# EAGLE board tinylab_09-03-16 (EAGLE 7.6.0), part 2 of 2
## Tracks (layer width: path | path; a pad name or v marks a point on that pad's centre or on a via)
3.3V  (via drill 0.51 pad 1.02)
  Top 0.406: 189.83,46.67 R37.2 | 189.83,40.96 R39.2 | v127.65,90.17 IC3.2 127.65,85.72
  Top 0.61: U$10.1 175.7,69.01 179.72,73.02 | Q4.1 189.83,40.96 | IC5.4 121.32,102.84 121.93,102.23 C12.A | 122.07,100.59 C12.A | 127.65,84.45 121.3,84.45 118.12,81.28 117.17,81.28 115.9,80.01 U$4.3V | 127.65,84.45 127.65,85.72 | 191.46,41.59 191.78,41.91 191.78,46.36 191.52,46.62 R37.2 189.19,47.31 187.02,47.31 186.38,46.67 Q3.1 185.7,49.26 185.43,49.53 185.43,69.21 185.7,69.48 C27.1 186.7,71.75 187.34,72.39 R42.2 R43.2 183.26,74.03 182.26,73.02 179.72,73.02 | 191.46,41.59 190.88,41.01 R39.2 | U5.4 198.06,30.41 v198.13,30.48 | 191.46,41.59 192.42,40.64 v192.42,39.37 192.1,39.05 177.49,39.05 175.27,36.83 C17.1 175.01,36.72 U$15.1 | 127.65,84.45 137.17,84.45 v140.35,87.63 | 179.72,73.02 178.13,74.61 178.13,83.5 177.49,84.14 JP8.3 JP8.5 JP8.6 171.15,86.68 170.51,86.04 170.51,82.23 171.15,81.6 JP8.2 | v127.65,100.33 127.33,100.65 125.74,100.65 125.43,100.96 124.52,100.96 C11.1 122.38,100.91 C12.A
  Bottom 0.61: v127.65,100.33 v127.65,90.17 | v198.13,30.48 198.13,35.56 196.23,37.47 194.32,37.47 v192.42,39.37 | v140.35,87.63 140.35,99.06 142.25,100.96 142.25,107.95 144.16,109.85 154.95,109.85 158.13,106.68 158.13,102.23 160.67,99.69 166.38,99.69 168.92,97.16 168.92,75.67 U$10.1
4  (via drill 0.51 pad 1.02, 0.6)
  Top 0.406: S11.4 156.22,62.23 U$4.D4 v144.79,62.23 | U$1.25 126.24,77.01 126.69,77.47 131.46,77.47 v132.09,76.83
  Bottom 0.406: v144.79,62.23 141.93,62.23 140.35,63.82 138.12,63.82 137.81,64.14 137.81,76.52 136.86,77.47 132.73,77.47 v132.09,76.83
5  (via drill 0.51 pad 1.02, 0.6)
  Top 0.406: U$1.31 121.44,81.42 122.57,82.55 135.27,82.55 135.9,81.91 135.9,80.64 136.54,80.01 139.08,80.01 v139.71,80.64 | S11.3 156.22,64.77 U$4.D5 v144.79,64.77
  Bottom 0.406: v139.71,80.64 139.71,78.74 139.08,78.1 139.08,65.41 139.71,64.77 v144.79,64.77
6
  Top 0.406: U$1.27 124.64,79.54 125.11,80.01 132.73,80.01 133.36,79.38 133.36,75.56 134,74.93 137.17,74.93 138.44,73.66 138.44,67.94 139.08,67.31 U$4.D6 156.22,67.31 S11.2
7  (via drill 0.51 pad 1.02, 0.6)
  Top 0.406: 118.21,62.78 v118.44,62.87 118.52,62.78 U$1.1 | v131.46,59.69 131.46,56.52 132.73,55.25 134,55.25 134.63,54.61 134.63,52.71 135.27,52.07 140.35,52.07 142.25,53.98 v142.25,55.88 | v142.25,60.96 v142.25,66.04 | S11.1 156.22,69.85 U$4.D7 v142.89,69.85
  Bottom 0.406: v131.46,59.69 130.19,58.42 126.38,58.42 124.47,56.52 119.39,56.52 118.44,57.47 v118.44,62.87 | v142.89,69.85 142.25,69.21 v142.25,66.04 | v142.25,55.88 v142.25,60.96
8
  Top 0.406: U$1.28 123.84,80.01 124.47,80.64 133.36,80.64 134,80.01 134,76.2 134.63,75.56 138.44,75.56 139.08,74.93 139.55,74.45 140.03,73.98 151.14,73.98 151.14,73.91 | U$4.D8 151.14,73.91 | 151.14,73.91 155.84,73.91 S12.10
9
  Top 0.406: U$1.29 123.04,80.48 123.84,81.28 134,81.28 134.63,80.64 134.63,78.74 135.58,77.79 147.33,77.79 148.6,76.52 150.44,76.52 U$4.D9 | U$4.D9 155.84,76.45 S12.9 | 150.51,76.52 U$4.D9
10
  Top 0.406: U$1.30 122.24,80.95 123.2,81.91 134.63,81.91 135.27,81.28 135.27,80.01 136.22,79.06 150.51,79.06 U$4.D10 155.84,78.99 S12.8
11  (via drill 0.51 pad 1.02, 0.6)
  Top 0.406: U$4.D11 151.14,81.53 | 151.14,81.53 155.84,81.53 S12.7 | v140.35,66.04 140.35,61.6 138.76,60.01 138.76,57.15 137.81,56.52 132.73,56.52 132.09,57.15 132.09,58.42 132.73,59.05 132.73,61.28 132.41,61.6 130.19,61.6 129.87,61.91 129.87,64.35 U$1.12 | v141.93,81.6 151.14,81.6 151.14,81.53
  Bottom 0.406: v141.93,81.6 140.98,80.64 140.98,66.67 v140.35,66.04
12  (via drill 0.51 pad 1.02, 0.6)
  Top 0.406: U$1.26 125.44,77.8 125.74,78.1 131.46,78.1 v132.41,78.74 | S12.6 155.84,84.07 U$4.D12 150.51,84.14 v141.3,84.14
  Bottom 0.406: v132.41,78.74 135.9,78.74 v141.3,84.14
13
  Top 0.406: U$1.32 120.64,81.89 121.93,83.19 137.81,83.19 141.3,86.68 151.08,86.68 151.14,86.61 | U$4.D13 151.14,86.61 | 151.14,86.61 155.84,86.61 S12.5
!RESET  (via drill 0.51 pad 1.02, 0.6)
  Top 0.406: S1.2 147.62,109.22 | 147.62,109.22 147.62,108.24 146.7,107.31 | 146.7,107.31 145.8,107.31 R48.1 | S1.1 147.62,106.39 146.7,107.31 | v133.36,57.79 134,58.42 134,62.23 133.68,62.55 131.77,62.55 131.14,63.18 131.14,65.09 130.82,65.41 129.66,65.41 U$1.13 | 120.03,52.07 J1.5 123.84,52.07 | 120.03,52.07 117.49,52.07 115.58,53.98 115.58,57.15 v116.22,57.79 | v126.38,107.31 126.38,107.95 v128.28,109.85 | v140.35,111.76 142.89,109.22 147.62,109.22 | v108.28,82.55 U$4.RESET | JP5.5 123.84,45.09 121.93,46.99 120.66,46.99 119.71,47.94 119.71,51.75 120.03,52.07
  Bottom 0.406: v133.36,57.79 127.01,57.79 125.11,55.88 J1.5 | 114.31,82.55 114.31,97.16 123.2,106.05 125.11,106.05 v126.38,107.31 | v128.28,109.85 130.82,109.85 132.73,107.95 132.73,104.14 133.36,103.5 139.71,103.5 140.98,104.77 140.98,111.12 v140.35,111.76 | 114.31,82.55 v108.28,82.55 | v116.22,57.79 115.58,58.42 115.58,81.28 114.31,82.55
+5V  (via drill 0.51 pad 1.02, 0.6, 1.02 pad 1.6)
  Top 0.406: R38.2 R40.2 | U$1.44 120.22,64.58 120.66,64.14 | 120.66,64.14 120.66,62.8 U$1.2 120.64,61.62 120.66,61.6 120.29,61.23 C4.2 | 125.43,72.39 120.66,72.39 120.47,72.58 U$1.34 110.31,72.58 105.42,77.47 U$4.5V | 125.43,72.39 126.38,72.39 127.01,73.02 127.01,74.35 U$1.24 | U$1.14 127.65,66.18 | 127.65,66.18 126.24,66.18 125.43,66.99 125.43,68.9 | v127.65,64.77 127.65,66.18 | 125.43,68.9 125.43,72.39 | R35.2 164.11,103.88 163.84,104.14 | R32.2 168.55,103.77 168.92,104.14 | v51.45,108.58 53.35,108.58 55.58,106.36 55.58,101.28 53.35,99.06 R45.2 | v151.78,12.06 151.96,12.24 151.78,12.24 | 120.66,64.14 120.66,65.41 124.16,68.9 125.43,68.9 | R13.2 46.95,107.37 v47,107.31
  Top 0.61: IC3.8 126.38,92.71 | IC3.8 126.38,92.08 123.25,92.08 Q2.2 | IC3.8 126.38,94.61 127.01,95.25 137.81,95.25 138.76,96.2 138.76,98.74 138.81,98.8 | C15.1 72.06,43.26 U$7.8 69.94,43.26 v69.23,43.18 | C25.1 80.92,43.55 v81.93,42.55 83.2,42.55 83.83,43.18 U2.8 | R19.1 7.37,14.34 7.63,14.61 18.43,14.61 | 18.43,14.61 23.51,14.61 24.41,13.71 R18.1 24.41,13.6 25.41,14.61 38.11,14.61 39.01,13.71 R12.2 39.01,13.6 40.02,14.61 45.1,14.61 45.73,13.97 45.73,12.06 | 45.73,12.06 C21.1 | 45.73,12.06 46.37,12.7 R11.2 52.45,13.71 53.35,14.61 55.26,14.61 56.53,13.33 56.53,12.06 57.16,11.43 61.61,11.43 62.24,10.79 62.24,3.17 63.83,1.59 69.32,1.59 70.5,2.77 MOTOR.1 70.52,5.11 72.43,5.11 74.04,3.49 79.07,3.49 82.56,6.98 v82.56,8.89 | 32.24,87.66 C14.A | C14.A 32.13,87.49 C13.1 32.13,78.47 26.68,70.48 | 26.68,70.48 26.68,66.67 25.41,65.41 20.33,65.41 19.06,64.14 19.06,50.8 | 19.06,50.8 19.06,49.53 18.43,48.9 v18.43,46.99 | v18.43,17.78 18.43,14.61 | C24.1 159.66,39.74 160.03,39.37 | 160.03,39.37 v161.94,39.37 | v161.94,29.21 161.94,34.93 161.3,35.56 159.47,35.56 158.84,36.11 SG2.+ 159.4,36.82 159.4,38.74 | v84.47,31.75 R27.1 82.83,34.03 81.93,34.93 v81.93,38.1 81.93,40.01 88.28,40.01 88.91,40.64 88.91,47.62 87.01,49.53 82.56,49.53 81.03,51.06 81.03,52.71 v71.13,52.71 | 159.4,38.74 160.03,39.37 | 20.33,51.07 C23.1 R46.2 30.23,51.07 30.49,50.8 30.49,47.62 31.76,46.36 38.75,46.36 40.02,47.62 IC6.19 | 20.33,51.07 19.33,51.07 19.06,50.8 | P1.E 162,12.96 163.84,11.11 163.84,8.26 162.57,6.98 | IC2.1 191.78,9.53 191.78,10.79 188.61,13.97 R24.2 183.79,15.61 183.53,15.88 177.81,15.88 176.54,14.61 176.54,10.16 173.37,6.98 162.57,6.98
  Top 0.61: 26.68,70.48 7.63,70.48 7.55,70.56 U$5.3 | R40.2 182.21,42.86 178.45,42.86 v177.49,43.82 | v19.06,93.34 20.65,91.76 32.4,91.76 | 32.4,91.76 IC4.18 | C14.A 32.27,91.63 32.4,91.76 | M1.2 20.97,33.97 20.33,34.61 20.33,51.07 | 162.57,6.98 v151.78,6.98 | 159.4,38.74 v157.49,38.74
  Top 0.813: C22.1 R15.2 184.21,87.05 185.11,87.95 185.11,89.22 | R16.2 R17.2 | R17.2 R14.2 | IC5.3 118.52,93.61 C10.A | C10.A 118.39,93.21 C5.2 118.39,89.16 118.12,88.9 111.14,88.9 109.23,90.8 | C10.A 120.03,93.34 120.4,93.71 C16.1 122.95,93.33 Q2.2 | 185.11,89.22 185.11,89.76 D2.C 185.02,89.95 | v156.86,104.14 163.84,104.14 168.92,104.14 173.05,104.14 175.27,101.92 175.27,98.72 K4.1 175.27,98.64 175.27,94.3 177.18,92.39 184.16,92.39 184.8,91.76 184.8,89.53 185.11,89.22 | v143.52,100.96 143.52,101.6 144.16,102.23 C26.1 | R48.2 145.43,104.14 144.16,104.14 143.52,103.5 v143.52,100.96 | v143.52,100.96 143.52,100.33 142.89,99.69 139.71,99.69 138.81,98.8 | R17.2 112.78,106.41 112.41,106.05 112.41,101.6 109.23,98.42 109.23,90.8 | v128.92,53.98 128.92,59.05 v128.28,59.69 | v151.78,24.77 v151.78,22.22 v151.78,19.68 v151.78,17.14 v151.78,14.61 151.78,12.24 v151.78,12.06 v151.78,9.53 v151.78,6.98 v151.78,4.45 v151.78,1.91 | JP5.1 134,45.09 133.36,45.72 130.82,45.72 130.19,46.36 J1.2 | 85.1,62.87 85.1,66.04 87.01,67.94 90.82,67.94 95.72,72.84 L2.2 U$4.5V | 85.1,62.87 85.1,56.78 81.03,52.71 | C30.+ 71.33,74.73 74.31,71.75 74.31,64.14 75.58,62.87 85.1,62.87 | 109.23,90.8 107.65,90.8 v106.69,89.85
  Top 1.016: IC1.4 92.52,80.67 L2.2
  Bottom 0.406: 31.13,108.58 47,108.58 | 47,108.58 v51.45,108.58 | v47,107.31 47,108.58
  Bottom 0.61: v81.93,42.55 v81.93,38.1 | U1.2 12.46,94.23 13.35,93.34 v19.06,93.34 25.41,93.34 26.05,93.98 26.05,103.5 31.13,108.58 | v18.43,46.99 v18.43,17.78 | v84.47,31.75 82.56,29.84 v82.56,8.89 | J1.2 131.46,49.53 132.09,50.17 132.09,53.34 130.82,54.61 129.55,54.61 v128.92,53.98 | JP5.1 134,41.28 134.63,40.64 147.33,40.64 149.24,38.74 154.32,38.74 154.64,38.42 157.18,38.42 v157.49,38.74 | v69.23,43.18 69.23,51.44 v71.13,52.71 | v161.94,29.21 161.94,20.32 | 161.94,20.32 161.94,20.22 | P1.E 162,20.26 161.94,20.32 | v161.94,39.37 169.56,39.37 170.19,40.01 BLUETOOTH.1 170.19,41.91 172.1,43.82 v177.49,43.82
  Bottom 0.813: v143.52,100.96 143.52,107.31 144.79,108.58 154.32,108.58 156.86,106.05 v156.86,104.14 | U$4.5V 105.74,77.47 106.69,78.42 v106.69,89.85 | v127.65,64.77 128.28,64.14 v128.28,59.69
A0  (via drill 0.51 pad 1.02)
  Top 0.406: S13.7 89.86,64.77 92.09,62.55 92.09,43.82 95.26,40.64 v97.17,40.64
  Bottom 0.406: P1.S 165.75,17.14 163.84,15.24 158.76,15.24 156.86,17.14 156.86,32.38 156.22,33.02 109.87,33.02 109.23,32.38 109.23,29.84 107.96,28.57 102.88,28.57 102.25,29.21 102.25,29.84 100.98,31.11 98.44,31.11 95.9,33.66 95.9,39.37 v97.17,40.64
A1  (via drill 0.51 pad 1.02)
  Top 0.406: v151.78,31.75 v151.78,37.47 | v163.21,38.1 R21.1
  Bottom 0.406: v151.78,31.75 151.14,32.38 110.5,32.38 109.87,31.75 109.87,29.21 108.6,27.94 102.25,27.94 101.61,28.57 101.61,29.21 100.34,30.48 97.8,30.48 95.26,33.02 95.26,48.26 92.09,51.44 92.09,61.6 91.45,62.23 S13.8 | v151.78,37.47 156.22,37.47 156.86,36.83 156.86,35.56 157.81,34.61 162.25,34.61 163.21,35.56 v163.21,38.1
A2
  Top 0.406: R24.1 181.99,9.06 R23.1
  Bottom 0.406: S13.9 90.18,59.69 91.45,58.42 91.45,50.8 94.63,47.62 94.63,32.38 97.17,29.84 99.71,29.84 100.98,28.57 100.98,27.94 101.61,27.3 109.23,27.3 110.5,28.57 110.5,31.11 111.14,31.75 149.87,31.75 156.22,25.4 156.22,16.51 158.13,14.61 176.45,14.61 R23.1
A3  (via drill 0.51 pad 1.02)
  Top 0.406: v97.8,28.57 101.61,28.57 102.25,27.94 111.14,27.94 v111.77,28.57
  Bottom 0.406: v97.8,28.57 97.17,29.21 96.53,29.21 93.99,31.75 93.99,46.99 90.82,50.17 90.82,55.88 89.55,57.15 S13.10 | v111.77,28.57 111.77,30.48 112.41,31.11 149.24,31.11 155.59,24.77 155.59,15.88 157.49,13.97 173.37,13.97 180.99,6.35 187.97,6.35 189.24,6.98 189.24,10.79 189.88,12.06 193.69,12.06 194.32,11.43 IC2.2
A4  (via drill 0.51 pad 1.02)
  Top 0.406: v95.9,27.3 98.44,27.3 99.07,27.94 100.98,27.94 101.61,27.3 112.41,27.3 v113.68,28.57 | v187.97,11.43 187.97,4.76 187.65,4.45 v184.16,4.45
  Top 0.61: v191.15,81.91 193.37,81.91 194,82.55 R25.1
  Bottom 0.406: v95.9,27.3 95.9,28.57 93.36,31.11 93.36,46.36 90.18,49.53 90.18,53.98 89.55,54.61 S13.11 | v113.68,28.57 113.68,29.84 114.31,30.48 148.6,30.48 154.95,24.13 154.95,15.24 156.86,13.33 172.73,13.33 181.62,4.45 v184.16,4.45 | v187.97,11.43 187.97,14.61 193.05,19.68 193.05,34.29 191.15,36.2 191.15,45.09 187.97,48.26 187.97,74.3 188.61,74.93 193.05,74.93 193.69,75.56 193.69,76.83 193.05,77.47 188.61,77.47 187.34,78.74 187.34,80.64 187.97,81.28 190.51,81.28 v191.15,81.91
A5  (via drill 0.51 pad 1.02)
  Top 0.406: S3.2 S3.1 S2.2 S2.1 58.35,5.37 R10.1 v59.7,5.08 | v87.64,6.98 88.28,7.62 88.28,11.43 87.01,12.7 83.83,12.7 83.16,12.11 81.29,10.24 81.29,8.89 80.06,7.66 SW1.P1 | S13.12 90.18,52.07 90.82,51.44 90.82,39.37 90.18,38.74 v89.55,38.74
  Bottom 0.406: v87.64,6.98 88.91,8.26 88.91,23.5 88.28,24.13 88.28,37.47 v89.55,38.74 | v59.7,5.08 61.46,5.08 63.54,7.16 78.24,7.16 SW1.P1
A_A0
  Top 0.406: U$1.36 113.54,70.98 111.14,68.58 111.14,65.41 110.5,64.77 U$4.A0 S13.6
A_A1
  Top 0.406: U$1.37 114.01,70.18 111.77,67.94 111.77,63.5 110.5,62.23 U$4.A1 S13.5
A_A2
  Top 0.406: U$1.38 114.48,69.38 112.41,67.31 112.41,60.96 111.14,59.69 U$4.A2 S13.4
A_A3
  Top 0.406: U$1.39 114.95,68.58 113.04,66.67 113.04,58.42 111.77,57.15 U$4.A3 S13.3
A_A4
  Top 0.406: U$1.40 115.42,67.78 113.68,66.04 113.68,55.88 112.41,54.61 U$4.A4 S13.2
A_A5
  Top 0.406: U$1.41 115.89,66.98 114.31,65.41 114.31,53.98 111.77,52.07 U$4.A5 S13.1
A_AREF  (via drill 0.51 pad 1.02)
  Top 0.406: U$1.42 116.36,66.18 114.95,64.77 114.95,62.23 115.95,61.23 C6.1 115.85,61.23 114.95,60.33 v114.95,52.07 | v113.68,81.28 v116.22,83.82 | v120.03,85.09 120.66,85.09 121.3,85.72 v125.74,85.72 | v128.92,85.72 134.63,85.72 140.35,91.44 150.25,91.44 U$4.AREF 155.84,91.69 S12.3
  Bottom 0.406: v114.95,52.07 114.95,80.01 v113.68,81.28 | v116.22,83.82 118.76,83.82 v120.03,85.09 | v125.74,85.72 v128.92,85.72
A_MISO  (via drill 0.51, 0.51 pad 1.02)
  Top 0.406: U$1.11 127.84,62.68 130.19,60.33 J1.1 131.46,52.07 132.09,51.44 132.09,47.62 132.73,46.99 134.63,46.99 v135.9,45.72 | JP5.2 131.46,40.64 130.82,40.01 118.76,40.01 118.12,40.64 118.12,43.82 117.49,44.45 113.04,44.45 110.5,46.99 S14.3 110.5,48.58 110.18,48.9 94.94,48.9 92.72,51.12 92.72,63.18 92.47,63.44 v92.47,67.72
  Bottom 0.406: v135.9,45.72 132.09,45.72 131.46,45.09 JP5.2 | v92.47,67.72 76.92,67.72 56.5,47.3 56.5,40.59 53.45,37.54 53.15,37.54 50.41,40.28 50.41,51.87 47.97,54.3 47.05,54.3 34.56,41.81 28.16,41.81 M1.7
A_MOSI  (via drill 0.51 pad 1.02)
  Top 0.406: U$1.10 127.04,57.12 v127.65,56.52 | J1.4 127.65,46.99 126.38,45.72 JP5.4 126.38,41.91 125.74,41.28 120.03,41.28 119.39,41.91 119.39,45.09 118.76,45.72 116.22,45.72 115.58,46.36 S14.1
  Bottom 0.406: J1.4 127.65,47.62 128.28,46.99 137.81,46.99 138.44,47.62 | 138.44,47.62 138.44,51.44 137.81,52.07 135.27,52.07 134,53.34 134,55.25 133.36,55.88 128.28,55.88 v127.65,56.52 | M1.6 25.41,39.68 23.89,41.2 23.89,53.09 40.65,69.85 40.65,72.29 53.44,85.08 61.28,85.08 85.74,109.54 85.74,114.3 87.01,115.57 96.74,115.57 97.04,115.27 151.9,115.27 170.8,96.37 170.8,75.64 177.2,69.24 177.2,50.34 175.76,48.9 171.15,48.9 169.89,47.64 169.89,44.55 169.28,43.94 155.56,43.94 151.9,47.6 138.49,47.6 138.44,47.62
A_RX  (via drill 0.51 pad 1.02)
  Top 0.406: U$1.20 131.32,70.98 132.73,72.39 v132.73,73.02 | U$4.D0 156.22,52.07 S11.8
  Bottom 0.406: v132.73,73.02 135.27,73.02 135.9,72.39 135.9,62.23 137.49,60.33 137.49,53.34 139.08,52.07 U$4.D0
A_SCK  (via drill 0.51, 0.51 pad 1.02)
  Top 0.406: U$1.9 126.24,55.39 127.33,54.29 | 127.33,54.29 127.65,53.98 J1.3 | JP5.3 128.92,41.28 128.28,40.64 119.39,40.64 118.76,41.28 118.76,44.45 118.12,45.09 114.31,45.09 113.04,46.36 S14.2 | v57.42,49.73 59.55,47.6 62.29,47.6 65.65,44.25 65.65,34.8 61.99,31.14 38.21,31.14 30.59,38.76 28.16,38.76 M1.5 | v104.71,78.68 115.84,78.68 116.54,79.38 117.41,79.38 v117.47,79.31 | v117.46,56.41 117.46,56.22 120.66,53.02 v122.57,53.02 123.84,54.29 127.33,54.29
  Bottom 0.406: v122.57,53.02 122.57,47.62 124.47,45.72 128.28,45.72 128.92,45.09 JP5.3 | v117.46,56.41 117.46,57.96 116.85,58.57 116.85,59.05 116.22,59.69 116.22,78.42 117.11,79.31 v117.47,79.31 | v104.71,78.68 104.47,78.92 104.47,88.27 102.57,90.17 101.3,90.17 99.39,88.27 99.39,84.45 98.12,83.19 91.45,83.19 58,49.73 v57.42,49.73
A_SCL  (via drill 0.51 pad 1.02)
  Top 0.406: U$1.18 130.99,69.38 131.46,69.85 132.73,69.85 133.36,70.48 v133.36,71.12 | v135.9,55.25 139.08,55.25 139.71,55.88 139.71,58.42 140.98,59.69 U$4.D3 156.22,59.69 S11.5 | U$4.SCL 155.84,96.77 S12.1
  Bottom 0.406: v133.36,71.12 134,71.12 134.63,70.48 134.63,61.6 136.54,59.69 136.54,55.88 v135.9,55.25 | U$4.D3 149.24,59.69 148.6,60.33 148.6,96.2 149.24,96.84 150.44,96.84 U$4.SCL
A_SDA  (via drill 0.51 pad 1.02, 0.6)
  Top 0.406: U$1.19 127.95,70.18 v127.65,70.48 | v135.9,53.34 139.08,53.34 140.98,55.25 140.98,56.52 141.62,57.15 U$4.D2 156.22,57.15 S11.6 | S12.2 155.84,94.23 U$4.SDA 150.25,93.98 v147.33,93.98
  Bottom 0.406: v127.65,70.48 132.09,70.48 133.36,69.21 133.36,60.96 135.9,58.42 135.9,56.83 135.27,56.2 134.95,56.2 134.63,55.88 134.63,54.61 v135.9,53.34 | v147.33,93.98 147.33,57.79 147.97,57.15 U$4.D2
A_TX  (via drill 0.51 pad 1.02)
  Top 0.406: U$1.21 130.85,71.78 131.46,72.39 v131.46,74.3 | U$4.D1 156.22,54.61 S11.7
  Bottom 0.406: v131.46,74.3 135.27,74.3 136.54,73.02 136.54,62.87 138.44,60.64 138.44,55.88 139.71,54.61 U$4.D1
D4  (via drill 0.51 pad 1.02)
  Top 0.406: v168.29,58.42 168.29,59.69 166.38,61.6 S11.13 | v164.48,46.36 163.21,45.09 154.32,45.09 v153.68,44.45 | v169.56,32.38 U$15.3 | v159.4,33.66 156.86,33.66 155.59,34.93 v155.59,39.69
  Bottom 0.305: 168.92,51.44 164.48,46.99
  Bottom 0.406: v168.29,58.42 168.92,57.79 168.92,51.44 | 164.48,46.99 v164.48,46.36 | v159.4,33.66 167.65,33.66 168.92,32.38 v169.56,32.38 | v153.68,44.45 155.59,42.55 v155.59,39.69
D5  (via drill 0.51 pad 1.02)
  Top 0.406: v169.56,59.69 168.92,60.33 168.92,63.5 168.29,64.14 S11.14 | v167.33,48.58 165.75,46.99 165.75,45.4 165.11,44.77 165.11,44.45 155.59,44.45 154.32,43.18 153.05,43.18 151.78,44.45 142.89,44.45 141.62,43.18 141.62,34.93 140.98,34.29 124.47,34.29 123.2,33.02 93.99,33.02 92.09,31.11 92.09,23.5 89.55,20.95 v89.55,1.27 | v60.34,13.33 64.41,13.33 R9.1
  Bottom 0.406: v169.56,59.69 169.56,50.8 v167.33,48.58 | v89.55,1.27 59.7,1.27 57.8,3.81 57.8,10.79 v60.34,13.33
D6  (via drill 0.51 pad 1.02)
  Top 0.406: v170.19,65.41 168.92,66.67 S11.15 | SW1.A 91.13,9.45 91.13,13.33 92.72,14.61 92.72,30.48 94.63,32.38 123.84,32.38 125.11,33.66 141.62,33.66 142.25,34.29 142.25,42.55 143.52,43.82 151.14,43.82 152.41,42.55 154.95,42.55 156.22,43.82 165.75,43.82 165.75,44.45 166.38,45.09 166.38,46.36 166.7,46.67 v167.33,46.67
  Bottom 0.305: 170.19,50.17 167.33,47.31 v167.33,46.67
  Bottom 0.406: v170.19,65.41 170.19,60.96 170.83,60.33 170.83,58.42 170.19,57.79 170.19,50.17
D7  (via drill 0.51 pad 1.02)
  Top 0.406: v172.1,67.94 170.83,69.21 S11.16 | v168.92,45.09 167.02,43.18 156.86,43.18 155.59,41.91 151.78,41.91 150.51,43.18 144.16,43.18 142.89,41.91 142.89,33.66 142.25,33.02 125.74,33.02 124.47,31.75 95.26,31.75 93.36,29.84 93.36,12.78 SW1.B
  Bottom 0.406: v172.1,67.94 172.1,58.42 170.83,57.15 170.83,49.53 168.92,47.62 v168.92,45.09
D8  (via drill 0.51 pad 1.02)
  Top 0.406: 22.87,9.87 S4.2 28.59,10.97 v28.59,12.06 | 22.87,9.87 S4.1 | R18.2 22.61,10.13 22.87,9.87 | v28.59,17.14 29.86,15.88 59.7,15.88 64.78,20.95 81.93,20.95 83.2,22.22 83.2,24.77 84.47,26.04 86.37,26.04 90.18,29.84 90.18,33.02 92.09,34.93 121.3,34.93 122.57,36.2 139.08,36.2 139.71,36.83 139.71,45.09 141.62,46.99 160.67,46.99 161.94,48.26 161.94,74.3 162.57,74.93 S12.11
  Bottom 0.406: v28.59,12.06 v28.59,17.14 28.59,22.54 27,24.13 21.6,24.13 20.97,24.77 20.97,30.8 21.6,31.43 31.13,31.43 32.08,32.38 32.08,35.56 31.13,36.51 M1.3
D9  (via drill 0.51 pad 1.02)
  Top 0.406: S5.2 9.54,9.87 | 9.54,9.87 7,9.87 | 7,9.87 S5.1 | R19.2 9.17,10.24 9.54,9.87 | 27.95,18.41 29.22,18.41 31.13,16.51 59.07,16.51 64.15,21.59 81.29,21.59 82.56,22.86 82.56,25.4 83.83,26.67 85.74,26.67 89.55,30.48 89.55,33.66 91.45,35.56 120.66,35.56 121.93,36.83 138.44,36.83 139.08,37.47 139.08,45.72 140.98,47.62 160.03,47.62 161.3,48.9 161.3,76.83 161.94,77.47 S12.12 | 27.95,18.41 26.68,17.14 21.6,17.14 19.7,19.05 17.16,19.05 15.25,17.14 7,17.14 6.36,16.51 6.36,11.43 7,10.79 7,9.87 | 27.95,18.41 27.95,19.05 v27.63,19.37
  Bottom 0.406: v27.63,19.37 27.63,22.22 26.68,23.18 20.65,23.18 20.01,23.81 20.01,35.88 20.65,36.51 M1.4
D10  (via drill 0.51 pad 1.02)
  Top 0.406: 59.7,22.22 80.66,22.22 81.93,23.5 81.93,26.04 83.2,27.3 85.1,27.3 88.91,31.11 88.91,34.29 90.82,36.2 120.03,36.2 121.3,37.47 137.81,37.47 138.44,38.1 138.44,46.36 140.35,48.26 159.4,48.26 160.67,49.53 160.67,79.38 161.3,80.01 S12.13 | v59.7,20.32 59.7,22.22 | R8.1 48.59,22.54 49.54,23.5 58.43,23.5 59.7,22.22
  Bottom 0.406: S6.3 62.88,34.93 59.7,31.75 v59.7,20.32
D11  (via drill 0.51 pad 1.02)
  Top 0.406: S12.14 160.67,82.55 160.03,81.91 160.03,50.17 158.76,48.9 139.71,48.9 137.81,46.99 137.81,38.74 137.17,38.1 120.66,38.1 119.39,36.83 90.18,36.83 88.28,34.93 88.28,31.75 84.47,27.94 82.56,27.94 81.29,26.67 81.29,24.13 80.02,22.86 60.34,22.86 55.89,27.3 45.73,27.3 v42.56,24.13 42.87,23.81 R7.1
  Bottom 0.406: S6.2 60.34,35.56 59.07,34.29 43.83,34.29 42.56,33.02 v42.56,24.13
D12  (via drill 0.51 pad 1.02)
  Top 0.406: 34.62,27.94 56.53,27.94 60.97,23.5 79.39,23.5 80.66,24.77 80.66,27.3 81.93,28.57 83.83,28.57 87.64,32.38 87.64,35.56 89.55,37.47 118.76,37.47 120.03,38.74 135.9,38.74 137.17,40.01 137.17,47.62 139.08,49.53 158.13,49.53 159.4,50.8 159.4,84.45 160.03,85.09 S12.15 | 34.62,27.94 26.31,27.94 R6.1 | v33.67,23.18 33.67,26.99 34.62,27.94
  Bottom 0.406: S6.1 56.53,36.83 55.26,35.56 41.29,35.56 38.75,33.02 38.75,28.26 v33.67,23.18
D13  (via drill 0.51 pad 1.02)
  Top 0.406: v141.62,92.71 137.81,92.71 136.22,94.3 132.41,94.3 131.52,93.41 IC3.5 | v156.86,102.23 156.86,101.6 159.4,99.06 159.4,88.9 160.67,87.63 S12.16
  Bottom 0.406: v141.62,92.71 141.62,97.79 142.25,98.42 143.52,98.42 144.79,99.69 144.79,104.77 145.43,105.41 152.41,105.41 154.95,102.87 156.22,102.87 v156.86,102.23
D+  (via drill 0.51 pad 1.02)
  Top 0.406: U$1.4 122.24,61.29 122.57,60.96 v122.57,59.05 | v128.28,104.77 v130.82,107.31 | R3.1 141.62,102.23 v140.35,100.96
  Bottom 0.406: v122.57,59.05 122.57,60.96 121.93,61.6 121.93,85.09 125.74,88.9 125.74,102.23 v128.28,104.77 | v130.82,107.31 130.82,103.5 131.46,102.87 138.44,102.87 v140.35,100.96
D-  (via drill 0.51 pad 1.02)
  Top 0.406: U$1.3 121.44,60.47 v121.3,60.33 | v127.01,106.05 v129.55,108.58 | v138.44,100.96 138.44,101.33 R2.1
  Bottom 0.406: v121.3,60.33 121.3,85.72 119.39,87.63 119.39,100.96 121.93,103.5 124.47,103.5 v127.01,106.05 | v129.55,108.58 129.55,106.68 130.19,106.05 130.19,102.87 131.46,101.6 137.81,101.6 v138.44,100.96
DB4
  Top 0.406: U1.11 35.32,109.79 40.02,105.09 40.02,98.74 39.38,98.11 37.07,98.11 IC4.13
DB5
  Top 0.406: IC4.14 37.07,96.84 40.33,96.84 40.97,97.47 40.97,106.68 37.86,109.79 U1.12
DB6
  Top 0.406: IC4.15 37.07,95.57 41.29,95.57 41.92,96.2 41.92,107.63 40.4,109.15 U1.13
DB7
  Top 0.406: IC4.16 37.07,94.3 42.24,94.3 42.94,95 U1.14
DIN  (via drill 0.51 pad 1.02)
  Top 0.406: R39.1 189.83,42.86 Q4.2 184.48,42.86 v184.16,42.55 | v184.8,72.39 184.16,71.75 184.16,68.58 183.53,67.94 179.72,67.94 176.67,64.89 U$10.3 174.83,64.89 173.68,66.04 173.68,76.83 175.27,78.42 JP8.1 | LED12.C 184.58,79.79 v182.89,78.1
  Bottom 0.406: v184.16,42.55 186.7,42.55 187.34,43.18 187.34,70.48 186.07,71.75 185.43,71.75 v184.8,72.39 182.89,74.3 v182.89,78.1
DOUT  (via drill 0.51 pad 1.02, 0.6)
  Top 0.406: U$10.2 176.13,66.89 v179.72,70.48 | 189.83,44.77 R37.1 | Q3.2 184.48,44.77 v184.16,44.45 | LED11.C 187.34,80.64 186.7,81.28 183.53,81.28 181.62,79.38 | 181.62,79.38 181.62,76.83 v180.99,76.2 | 181.62,79.38 181.62,83.19 178.13,86.68 178.13,90.49 177.49,91.12 173.37,91.12 172.73,90.49 JP8.8
  Top 0.61: Q3.2 186.06,44.77 186.7,44.13 189.19,44.13 R37.1
  Bottom 0.406: v184.16,44.45 186.07,44.45 186.7,45.09 186.7,68.58 184.8,70.48 v179.72,70.48 178.45,71.75 178.45,73.66 v180.99,76.2
E  (via drill 0.51 pad 1.02)
  Top 0.406: v22.87,97.79 24.46,99.38 36.94,99.38 IC4.12
  Bottom 0.406: v22.87,97.79 22.62,98.04 U1.6
GND  (via drill 0.51 pad 1.02, 1.02 pad 1.6)
  Top 0.406: LED6.K 54.62,19.05 53.99,18.41 41.29,18.41 | 41.29,18.41 40.02,19.68 40.02,20.32 LED5.K | 41.29,18.41 32.4,18.41 29.86,20.95 LED4.K 24.78,19.68 23.51,18.41 22.24,18.41 20.97,19.68 12.08,19.68 10.81,20.95 LED3.K | v80.34,36.51 80.02,36.51 79.07,37.47 79.07,37.78 78.36,37.78 U$7.4 | 174.76,51.56 174.77,51.69 | 182.38,59.49 182.41,59.47 | 127.96,74.3 127.88,74.38 U$1.23 127.96,74.51 127.96,76.2 130.51,76.2 130.82,75.88 v130.82,75.56 | U$1.35 118.06,71.75 119.39,71.75 120.03,71.12 v120.03,69.21 120.03,65.38 U$1.43 | v124.16,66.67 123.04,66.67 U$1.5 | v127.33,67.94 128.3,66.98 U$1.15
  Top 0.61: U1.1 9.92,112.78 10.81,113.66 19.06,113.66 20.08,112.64 U1.5
  Top 0.813: v100.98,24.77 v100.98,22.22 | v100.98,19.68 v100.98,17.14 v100.98,14.61 v100.98,12.06 100.98,10.16 | 100.98,10.16 v100.98,9.53 v100.98,6.98 v100.98,4.45 v100.98,1.91 | 150.44,89.22 U$4.GND | SW1.C 100.98,10.16
  other vias: 36.52,80.64 42.56,80.33 80.02,42.23 84.78,46.99 144.16,88.9 113.99,104.77 117.17,104.77 118.12,53.66 136.85,96.52 97.17,96.52 97.17,93.34 97.17,90.17 84.47,90.17 84.47,93.34 84.47,96.52 87.32,100.65 91.13,100.65 94.31,100.65 24.14,84.77 135.27,49.53 66.37,17.78 45.73,20.64 30.49,25.08 36.84,38.1 15.25,33.97 8.9,55.56 65.42,95.88 167.33,76.52 198.77,20 187.02,18.1 155.27,4.76 133.36,28.26 146.06,37.78 117.8,49.85 96.85,47.62 173.05,55.88 165.11,36.2 173.68,45.4 170.83,45.4 139.08,62.23 140.98,58.1 77.8,50.17 75.89,56.52 65.42,61.6 96.21,21.27 68.27,30.16 85.1,34.61 154.32,105.73 198.13,76.52 4.14,92.08 20.65,74.93 13.35,19.68 16.2,8.89 31.44,7.62 55.26,32.38 65.1,101.6 169.24,71.75 196.23,45.72 147.01,50.8 132.09,65.72 133.04,93.03 137.81,105.09 127.96,113.66 90.18,76.52 150.19,100.65 97.48,68.26 84.47,52.07 55.89,49.21 171.78,78.1 181.3,88.27 175.59,74.93 117.8,19.68 106.37,4.45 144.47,3.49 144.79,27.94 106.37,24.13 112.09,12.7 126.38,9.21 132.09,20.64 120.98,12.38 137.49,12.06 116.85,4.13 134,3.49 125.11,24.45 109.87,19.05 142.57,19.05 47.32,103.19 54.62,110.81 53.35,103.82 120.98,54.61 134.95,57.47 144.16,53.34 153.05,40.32 161.62,37.15 169.56,34.29 182.89,30.48 21.92,46.04 155.59,71.75 144.47,72.07 107.64,72.39 142.89,75.25 136.22,76.52 64.46,9.53 27.95,55.25 48.91,70.17 26.05,58.1 112.09,84.45 115.58,87.31 136.85,73.98 127.65,76.2 133.36,87.95 137.17,86.68 124.15,70.8 127.33,79.06 130.82,79.06 109.55,76.52 105.1,73.66 100.34,73.66 118.44,74.3 120.98,49.85 174,42.55 180.35,44.77 175.27,38.74 39.06,65.72 13.03,15.88 20.01,16.19 48.59,14.29 64.78,32.38 14.3,28.26 91.13,17.78 144.47,80.33 143.84,85.41 107.33,53.34 107.33,55.88 107.33,58.42 107.33,60.96 107.33,63.5 181.62,71.75 191.46,88.27 134.95,113.35 136.85,113.35 138.76,113.35 79.39,65.09 154,90.17 172.1,51.44 182.26,69.21 81.29,29.53 162.89,107.31 160.67,102.55 121.93,107.63 113.04,93.34 124.79,93.34 130.5,98.42
  pour Top (isolate 0.305): 80.02,40.64 71.77,40.64 71.77,24.77 78.12,24.77 78.12,33.02 80.02,33.02
  pour Bottom (isolate 0.406): 6.49,117.16 194.51,117.16 arc-90 201.31,109.41 201.31,6.3 arc-90 195,0 6.31,0 arc-90 0.01,6.3 0.01,110.04 arc-90
  pour Top (isolate 0.406): 6.23,117.16 194.12,117.16 arc-90 201.31,109.34 201.31,6.29 arc-90 195.02,0 6.3,0 arc-90 0.01,6.29 0.01,109.67 arc-90
LED
  Top 0.406: U$15.10 181.62,27.3 186.07,22.86 R33.2
LIGHT
  Top 0.406: IC4.17 37.04,93.03 42.24,93.03 43.83,94.61 43.83,105.41 44.09,105.67 R31.2
MISO  (via drill 0.51 pad 1.02)
  Top 0.406: v107.33,30.48 107.96,31.11 125.11,31.11 126.38,32.38 149.24,32.38 151.78,29.84 153.68,29.84 157.49,26.04 171.46,26.04 173.37,24.13 173.37,22.22 174,21.59 v182.89,21.59 | v189.24,26.67 193.69,26.67 194.12,27.11 U5.7
  Bottom 0.406: v107.33,30.48 107.33,39.37 107.96,40.01 S14.4 | v182.89,21.59 184.16,21.59 v189.24,26.67
MOSI  (via drill 0.51 pad 1.02)
  Top 0.406: v103.52,30.48 103.52,29.21 104.15,28.57 109.23,28.57 110.5,29.84 126.38,29.84 127.65,31.11 147.97,31.11 150.51,28.57 152.41,28.57 156.86,24.13 v167.65,24.13 | v172.73,27.3 172.73,29.21 173.37,29.84 U$15.5
  Bottom 0.406: v167.65,24.13 169.56,24.13 v172.73,27.3 | S14.6 115.58,41.91 114.31,43.18 105.1,43.18 104.47,42.55 104.47,32.7 103.52,31.75 v103.52,30.48
N$1
  Top 0.406: U$3.D- 139.06,105.06 R2.2
N$2
  Top 0.406: U$3.D+ 140.98,109.85 141.62,109.22 R3.2
N$3
  Top 0.406: LED3.A 7.37,21.32 7.37,23.86 8.9,25.4 R1.2
N$4
  Top 0.406: U$1.6 123.84,57.28 C1.2
N$5
  Top 0.406: S2.4 54.62,9.87 | 54.62,9.87 S2.3 | R11.1 54.25,10.24 54.62,9.87
N$6
  Top 0.406: C3.2 137.05,63.75 Y1.1 137.17,66.21 137.17,67.31 136.54,67.94 134,67.94 132.73,67.31 R4.1 131.99,67.78 U$1.16
N$7
  Top 0.406: C2.2 134.75,72.14 Y1.3 133.68,69.8 R4.2 132.46,68.58 U$1.17
N$8
  Top 0.406: T2.B 167.6,37.78 R21.2 167.28,37.1 167.02,36.83 R22.2
N$9
  Top 0.406: U$1.33 119.84,75.12 119.02,75.94 R5.1
N$10
  Top 1.016: IC1.2 89.12,83.19 | 89.12,83.19 89.12,80.67 L2.1 | D1.C 81.93,85.09 83.83,83.19 89.12,83.19
N$11
  Top 0.406: S3.4 36.84,9.87 | 36.84,9.87 S3.3 | R12.1 37.21,10.24 36.84,9.87
N$12
  Top 0.406: R9.2 R20.2 67.76,11.6
  Top 0.61: 67.76,11.6 69.14,11.6 T1.B
N$13
  Top 0.406: R6.2 22.61,21.32 LED4.A
N$14
  Top 1.676: JP1.3 195.75,98.42 195.91,98.42 195.27,99.06 193.37,99.06 188.61,103.82 178.13,103.82 175.27,106.68 175.27,110.83 K4.O
N$15
  Top 0.406: 37.21,21.32 LED5.A 36.84,22.54 37.48,23.18 40.97,23.18 41.29,22.86 41.29,20.64 41.87,20.05 R7.2
N$16
  Top 0.61: T1.C 72.66,14.33 73.67,13.31 73.67,7.62 73.04,6.98 67.4,6.98 MOTOR.2
N$17
  Top 0.406: 52.45,21.32 LED6.A 51.18,20.05 R8.2
N$18  (via drill 0.51 pad 1.02)
  Top 0.406: T2.C 171.29,35.1 171.46,34.93 171.78,34.93 v172.1,34.61
  Bottom 0.406: SG2.- 158.76,29.84 159.4,30.48 170.19,30.48 171.46,31.75 171.46,33.97 v172.1,34.61
N$19
  Top 0.406: LED1.A R15.1
N$20
  Top 0.406: R26.2 R25.2
  Top 0.61: T3.B 195.42,86.83 194.96,86.36 194.06,86.36 R25.2
N$21
  Top 0.406: LED1.C 189.98,88.9 D2.A
  Top 0.813: 192.74,89.85 T3.C 193.37,90 | 192.74,89.85 D2.A | 192.74,89.85 193.05,90.17 193.05,93.34 192.1,94.3 188.93,94.3 187.34,95.88 187.34,98.64 K4.2
N$22
  Top 0.406: R14.1 LED2.A
N$23
  Top 0.406: R17.1 LED8.A
N$24
  Bottom 1.676: JP1.2 195.51,103.5 183.53,103.5 181.3,101.28 K4.P
N$25
  Bottom 1.676: JP1.1 189.59,108.58 K4.S
N$26
  Top 1.676: J2.PWR 107.96,101.6 | 99.07,106.36 97.17,108.27 91.45,108.27 90.82,108.9 91.13,108.9 S9.2
  Top 1.778: 99.07,106.36 104.15,101.28 107.65,101.28 107.96,101.6
N$27
  Top 0.406: Q1.3 80.66,107 81.29,107.63 85.64,107.63 LED13.C
  Top 1.676: Q1.3 81.08,103.89 S9.3
N$29
  Top 0.406: R28.1 48.27,97.16 47.96,96.84 IC4.5
N$30
  Top 0.406: R29.1 48.59,95.25 48.27,95.57 IC4.4
N$31
  Top 0.406: R30.1 48.59,93.34 47.64,94.3 IC4.3
N$32  (via drill 0.6)
  Top 0.406: R27.2 v79.39,31.75
  Bottom 0.406: SW1.P2 78.74,17.77 80.02,19.05 80.02,29.21 79.39,29.84 v79.39,31.75
N$33
  Top 0.406: R44.1 48.59,101.65 T4.B 48.11,104.46 46.69,104.46 46.1,103.88 R31.1
N$34
  Top 0.406: U$5.2 6.36,74.21 6.36,91.44 15.25,100.33 15.25,111.13 U1.3
N$35
  Top 0.406: U1.16 48.27,111.13 48.27,108.41 T4.C
N$36
  Top 0.305: U$7.2 75.58,36.2 U$9.1
N$37  (via drill 0.51 pad 1.02)
  Top 0.61: v78.75,34.93 76.85,36.83 U$7.3 | v67.96,26.67 65.42,29.21 27.32,29.21 26.05,30.48 7.32,30.48 U$6.+$1
  Bottom 0.61: v67.96,26.67 76.21,26.67 78.12,28.57 78.12,34.29 v78.75,34.93
N$38
  Top 0.61: IC6.14 46.37,48.26 47,47.62 49.54,47.62 50.18,48.26 50.18,59.05 47.64,61.6 37.48,61.6 34.3,64.77 U$13.11
N$39
  Top 0.406: U$15.4 177.18,31.11 177.81,31.75 177.81,36.83 178.45,37.47 186.07,37.47 188.61,34.93 188.61,32.38 189.49,31.5 U5.3
N$40
  Top 0.406: U$15.6 177.18,28.57 179.08,30.48 179.08,36.2 179.72,36.83 185.43,36.83 187.34,34.93 187.34,31.11 189.15,29.3 U5.5
N$41
  Top 0.305: U$7.1 74.31,36.2 U$9.2
N$42
  Top 0.406: LED9.A R33.1
N$43  (via drill 0.51 pad 1.02)
  Top 0.406: U$15.2 175.91,33.66 176.54,34.29 176.54,36.83 177.81,38.1 186.7,38.1 189.88,34.93 189.88,33.66 190.93,32.61 193.05,32.61 | U5.2 193.05,32.61 | LED9.C 195.59,22.86 v196.23,22.22 | v194.32,36.2 194.32,35.56 193.05,34.29 193.05,32.61
  Bottom 0.406: v196.23,22.22 196.23,34.29 v194.32,36.2
N$44
  Top 0.813: L1.1 135.73,104.6 136.54,105.41 136.58,107.85 U$3.VBUS
N$45
  Top 0.406: R36.2 R34.1 C18.1 131.83,90.17 129.55,90.17 128.92,89.53 IC3.3
N$46
  Top 0.406: R41.1 LED10.A
N$47
  Top 0.406: IC3.1 123.26,88.2 122.95,88.52 Q2.3
N$48  (via drill 0.51 pad 1.02)
  Top 0.406: IC3.6 IC3.7 127.65,92.08 126.38,90.8 125.11,90.8 v124.47,90.17 | v111.77,81.28 111.77,81.91 115.58,85.72 v116.22,85.72 | v121.93,86.99 121.3,86.99 120.66,86.36 v118.76,86.36 | v28.9,30.48 64.78,30.48 67.32,33.02 v67.32,41.91 | v24.78,28.89 22.87,28.89 19.38,25.4 R1.1
  Bottom 0.406: v111.77,81.28 112.41,80.64 112.41,80.01 113.04,79.38 113.04,69.21 110.5,66.67 85.74,66.67 80.02,60.96 71.13,60.96 67.96,57.79 67.96,45.09 67.32,44.45 v67.32,41.91 | v124.47,90.17 124.47,89.53 v121.93,86.99 | v116.22,85.72 117.17,85.72 117.8,86.36 v118.76,86.36 | v28.9,30.48 28.9,29.53 28.27,28.89 v24.78,28.89
N$49
  Top 0.406: R42.1 LED11.A
N$50
  Top 0.406: R43.1 LED12.A
N$51
  Top 0.406: R47.2 73.67,107.63 75.58,109.54 85.64,109.54 LED13.A
N$52
  Top 0.406: R45.1 48.91,99.06 47.96,98.11 IC4.6
N$53
  Top 0.61: R46.1 28.59,46.36 29.86,45.09 39.38,45.09 41.29,46.99 IC6.18
N$54
  Top 0.61: IC6.16 43.83,45.72 44.46,45.09 50.81,45.09 52.72,46.99 52.72,62.23 50.81,64.14 45.73,64.14 44.46,65.41 U$13.7
N$55
  Top 0.61: IC6.20 38.75,52.71 39.38,53.34 U$13.4
N$56
  Top 0.61: IC6.23 34.94,52.71 34.3,53.34 U$13.2
N$57
  Top 0.61: IC6.21 37.48,48.26 36.84,47.62 33.03,47.62 31.76,48.9 U$13.1
N$58
  Top 0.61: IC6.15 45.1,46.99 45.73,46.36 50.18,46.36 51.45,47.62 51.45,60.33 48.91,62.87 39.38,62.87 36.84,65.41 U$13.10
N$59
  Top 0.61: IC6.17 42.56,52.71 41.92,53.34 U$13.5
N$60
  Top 0.61: IC6.22 36.21,52.71 36.84,53.34 U$13.3
N$61  (via drill 0.51 pad 1.02)
  Top 0.61: IC6.7 41.29,38.74 41.92,38.1 48.91,38.1 v51.45,40.64
  Bottom 0.61: v51.45,40.64 51.45,53.34 48.91,55.88 U$13.6
N$62  (via drill 0.51 pad 1.02)
  Top 0.61: IC6.6 40.02,37.47 41.29,36.2 50.81,36.2 v53.35,38.74
  Bottom 0.61: v53.35,38.74 53.35,53.98 41.92,65.41 U$13.8
N$63
  Top 0.61: IC6.11 46.37,43.18 47,43.82 51.45,43.82 53.99,46.36 53.99,72.39 52.08,74.3 40.02,74.3 39.38,73.66 U$13.9
N$64  (via drill 0.51 pad 1.02)
  Top 0.61: IC6.2 34.94,43.18 34.3,43.82 29.22,43.82 25.73,47.31 24.14,47.31 v22.87,48.58
  Bottom 0.61: v22.87,48.58 22.87,57.79 31.76,66.67 U$13.12
N$65
  Top 0.406: R13.1 45.1,111 U1.15
N$119
  Top 0.406: R16.1 LED7.A
RS
  Top 0.406: U1.4 17.54,103.12 20.01,100.65 36.94,100.65 IC4.11
RSSI  (via drill 0.51 pad 1.02, 0.6)
  Top 0.406: R41.2 190.25,74.03 191.15,74.93 191.15,75.56 v191.78,76.2 | U$10.6 180.83,58.9 181.62,59.69 v181.62,60.33
  Bottom 0.406: v191.78,76.2 187.34,76.2 184.16,79.38 180.35,79.38 179.72,78.74 179.72,76.2 177.18,73.66 177.18,71.12 177.81,70.48 177.81,61.6 178.77,60.64 181.3,60.64 v181.62,60.33
RX  (via drill 0.51 pad 1.02)
  Top 0.406: Q3.3 183.16,45.72 R38.1 178.82,46.62 v178.77,46.67 | v172.73,39.37 165.75,39.37 165.11,40.01 BLUETOOTH.3 | S11.9 166.38,51.44 v170.83,46.99
  Bottom 0.406: v170.83,46.99 178.45,46.99 v178.77,46.67 178.77,42.23 178.45,41.91 176.86,41.91 174.32,39.37 v172.73,39.37
RXLED  (via drill 0.51 pad 1.02)
  Top 0.406: U$1.8 125.44,64.47 v125.74,64.77 | v128.28,102.87 125.11,106.05 125.11,113.66 124.69,114.08 LED2.C
  Bottom 0.406: v125.74,64.77 123.2,64.77 122.57,65.41 122.57,84.45 126.38,88.27 126.38,100.96 v128.28,102.87
S_D10
  Top 0.406: S6.4 62.88,41.91 64.78,40.01 64.78,34.93 63.51,33.66 36.84,33.66 33.67,36.83 IC6.1
S_D11
  Top 0.406: S6.5 60.34,42.55 59.7,41.91 48.43,41.91 IC6.12
S_D12  (via drill 0.51 pad 1.02)
  Top 0.406: IC6.13 v47.64,53.34
  Bottom 0.406: v47.64,53.34 47.64,38.1 48.91,36.83 53.99,36.83 57.8,40.64 S6.6
SCK  (via drill 0.51 pad 1.02)
  Top 0.406: v105.42,30.48 105.42,29.84 106.06,29.21 108.6,29.21 109.87,30.48 125.74,30.48 127.01,31.75 148.6,31.75 151.14,29.21 153.05,29.21 156.86,25.4 170.83,25.4 172.73,23.5 172.73,21.59 173.37,20.95 175.91,20.95 v177.18,19.68 | v177.18,24.13 177.18,26.04 | 177.18,26.04 177.18,26.67 176.54,27.3 U$15.7 | U$15.9 177.18,26.04
  Bottom 0.406: v105.42,30.48 105.42,41.91 106.06,42.55 111.77,42.55 113.04,41.28 S14.5 | v177.18,19.68 v177.18,24.13
SCL  (via drill 0.51 pad 1.02)
  Top 0.406: U2.6 86.37,41.91 85.74,41.28 77.48,41.28 76.85,41.91 U$7.6 76.85,45.72 v74.94,45.72 74.94,46.99 73.67,48.26 60.34,48.26 56.53,52.07 56.53,82.23 52.4,86.36 52.4,88.9 49.54,91.76 IC4.1 | v89.55,26.35 90.82,27.3 90.82,32.38 92.72,34.29 121.93,34.29 123.2,35.56 139.71,35.56 140.35,36.2 140.35,44.45 142.25,46.36 161.3,46.36 162.57,47.62 162.57,58.42 163.21,59.05 S11.12 | R35.1 162.31,98.05 162.57,97.79 S12.20
  Bottom 0.406: v74.94,45.72 76.85,43.82 90.18,43.82 90.82,43.18 90.82,27.3 v89.55,26.35 | S12.20 162.57,97.79 160.67,95.88 160.67,60.33 161.94,59.05 S11.12
SDA  (via drill 0.51 pad 1.02)
  Top 0.406: U$7.5 78.12,48.26 | 78.12,48.26 82.56,48.26 | 82.56,48.26 86.37,48.26 87.64,46.99 U2.5 | v167.65,55.88 167.02,56.52 S11.11 | v165.11,49.53 165.11,48.9 161.94,45.72 142.89,45.72 140.98,43.82 140.98,35.56 140.35,34.93 123.84,34.93 122.57,33.66 93.36,33.66 91.45,31.75 91.45,25.4 v90.82,24.77 | v82.56,45.09 82.56,48.26 | 78.12,48.26 76.21,48.26 74.94,49.53 60.97,49.53 57.8,52.71 57.8,85.72 v57.16,86.36 | R32.1 166.75,99.33 167.65,98.42 167.65,95.88 167.02,95.25 S12.19 | IC4.2 43.51,93.03 43.19,92.71 43.19,85.09 43.83,84.45 v48.91,84.45
  Bottom 0.406: v167.65,55.88 167.65,51.44 165.75,49.53 v165.11,49.53 | v82.56,45.09 83.2,45.72 91.45,45.72 92.09,45.09 92.09,33.02 91.45,32.38 91.45,25.4 v90.82,24.77 | v57.16,86.36 50.81,86.36 v48.91,84.45 | S12.19 162.57,95.25 161.3,93.98 161.3,73.66 163.21,71.75 165.75,71.75 167.65,69.85 167.65,60.96 167.02,60.33 167.02,57.79 165.75,56.52 S11.11
TX  (via drill 0.6)
  Top 0.406: Q4.3 185.43,41.74 185.43,41.28 185.17,41.01 R40.1 182.21,40.96 178.13,40.96 177.49,41.59 177.49,41.91 175.27,44.13 173.05,44.13 v172.1,45.09 | 172.42,44.77 v172.1,45.09 | S11.10 172.73,53.98 173.37,53.34 173.37,47.62 172.1,46.36 v172.1,45.09
  Bottom 0.406: v172.1,45.09 171.46,44.45 170.83,44.45 169.56,43.18 163.21,43.18 162.57,42.55 BLUETOOTH.4
TXLED  (via drill 0.51 pad 1.02)
  Top 0.406: U$1.22 129.64,74.84 v129.55,74.93 | v121.93,109.85 121.93,113.66 121.52,114.08 LED8.C
  Bottom 0.406: v129.55,74.93 129.55,83.82 130.19,84.45 130.19,86.36 129.55,86.99 129.55,94.61 128.6,95.57 128.6,100.01 129.55,100.96 129.55,105.41 126.38,109.22 122.57,109.22 v121.93,109.85
VCC  (via drill 0.51 pad 1.02)
  Top 0.406: v109.87,81.28 109.87,84.45 111.77,86.36 v111.77,86.99 | R36.1 138.18,91.7 v138.44,91.44 | v119.71,104.77 122.88,104.77 126.06,101.6 129.87,101.6 130.51,100.96 v130.51,100.33
  Top 0.813: v87.64,69.85 v85.74,69.85 83.83,69.85 80.8,72.88 C28.+
  Top 1.016: Q1.2 82.94,88.9 | 82.94,88.9 82.94,87.89 84.47,86.36 87.34,86.36 IC1.1 | C28.+ 78.89,72.88 72.4,79.38 72.4,87.63 73.67,88.9 82.94,88.9
  Bottom 0.406: v109.87,81.28 109.87,80.01 111.77,78.1 111.77,71.75 109.87,69.85 U$4.VIN | v111.77,86.99 111.77,97.79 116.85,102.87 117.8,102.87 v119.71,104.77 | v138.44,91.44 132.09,91.44 130.82,92.71 130.82,94.3 129.24,95.88 129.24,99.06 v130.51,100.33
  Bottom 0.813: U$4.VIN v87.64,69.85 v85.74,69.85
VUSB  (via drill 0.51 pad 1.02)
  Top 0.406: U$1.7 124.64,60.8 125.11,60.33
  Top 0.813: L1.2 133.53,102.41 132.73,101.6 132.68,99.78 C20.A 132.46,99.56 C19.1 132.46,96.89 124.52,96.89 v124.47,96.84 | v117.49,82.55 117.49,86.99 118.12,87.63 120.03,87.63 v120.66,88.27 120.92,88.52 Q2.1 | v125.11,59.05 125.11,60.33
  Bottom 0.813: v120.66,88.27 120.66,95.25 122.25,96.84 v124.47,96.84 | v125.11,59.05 123.84,57.79 120.66,57.79 119.39,59.05 119.39,60.96 120.03,61.6 120.03,63.82 119.39,64.45 118.44,64.45 117.17,65.72 117.17,75.88 119.71,78.42 119.71,80.33 v117.49,82.55

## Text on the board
tPlace: RESET | 7-12V | ON | TX | RX | Fault | NO | POWER IN | ON | COM | RELAY | (Pin A4) | NC | ESP8266 | TX | RX | RSSI | 16x2 LCD | LCD CONTRAST | (Address 0x20) | 3.3V | DIO0 | DOUT | DIO1 | DIN | DIO2 | 7-SEGMENT | DIO3 | DIO12 | Din=Pin D10 | RST | XBee | RTS | CLK=Pin D12 | Load=Pin D11 | RSSI | DIO5 | ( | ) | DIO11 | RES | RES | DIO9 | RESET | SCK | MISO | DTR | CTS | ICSP | GND | DIO4 | RTC BATTERY | To Control 7-Segment | 5V | GND | MOSI | TX | RX | GND | 5V | SD CARD | BLUETOOTH | (CS=Pin D4) | RTC | EEPROM | 5V | GND | MOSI | SCK | MISO | (Address 0x68) | (Address 0x50) | RESET | To Control LEDs | BUZZER | (Pin A1) | GND | 5V | ROTARY ENCODER | A=Pin D6 | B=Pin D7 | Button=Pin A5 | ( | ) | L1 | L2 | L3 | L4 | (Pin D13) | (Pin D12) | (Pin D11) | (Pin 10) | 5V | GND | MOTOR | (Pin D5) | (Pin A2) | (Pin A3) | TEMPERATURE | PHOTORESISTOR | S1 | S2 | S3 | S4 | POTENTIOMETER | (Pin D9) | (Pin D8) | (Pin A5 low) | (Pin A5 high) | (Pin A0) | v2 | 07-11-16
anno: Released under the GNU-GPL v2 | https://www.tinylab.cc | Designed by: Yusuf Gundogdu | Revised by: Okan Saracoglu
